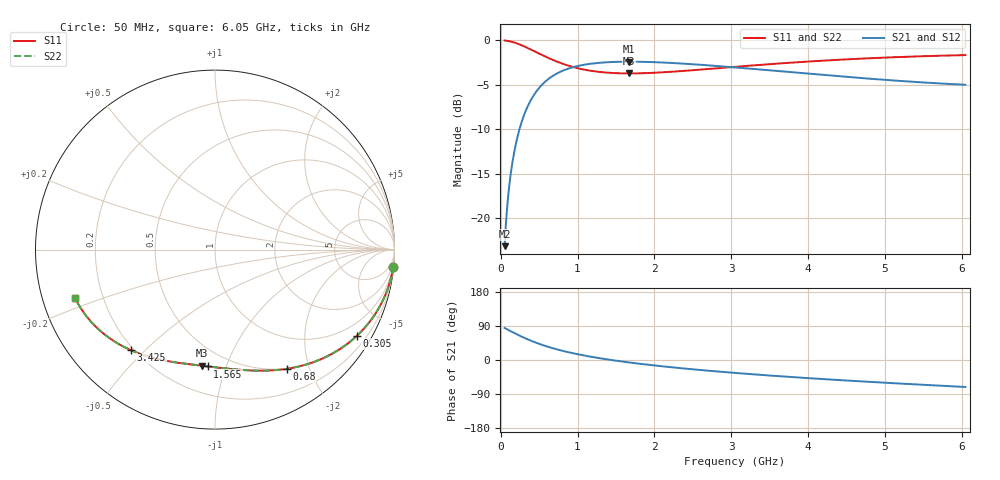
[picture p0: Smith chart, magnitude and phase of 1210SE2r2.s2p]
! AVX Thin Film Operation		Date: August 2001
! Description: Accu-P® Series, Thin Film, SMD, RF Capacitor
! Part Number: 12101J2R2ABT
! 50 MHz  -  6.05 GHz
! Serial Measurements
# mhz S db R 50
!	S11		S21		S12		S22
!	dB	Phase	dB	Phase	dB	Phase	dB	Phase
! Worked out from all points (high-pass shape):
!   401 points, 50 MHz to 6.05 GHz, reference 50 ohm
!   highest |S21| = -2.40 dB at 1.67 GHz (marker M1); lowest = -23.1 dB at 50 MHz (marker M2)
!   |S21| within 3 dB of the highest: 494.6 MHz to end of sweep
!   lowest |S11| = -3.7 dB at 1.67 GHz (marker M3), VSWR 4.74, Z = 18.3 - j41.2 ohm
!   |S11| at or under -10 dB: nowhere
!   |S22| runs from -3.7 to 0.0 dB; largest |S21 - S12| = 0
!   S11 on the Smith chart (normalised r, x): 50 MHz: 1, -21; 305 MHz: 0.53, -3.48; 680 MHz: 0.50, -1.65; 1.565 GHz: 0.38, -0.86; 3.425 GHz: 0.19, -0.45; 6.05 GHz: 0.10, -0.16
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50  -0.02 -5.5  -23.12 84.5  -23.12 84.5  -0.02 -5.5
65  -0.04 -7.1  -20.86 82.9  -20.86 82.9  -0.04 -7.1
110  -0.10 -12.0  -16.38 78.0  -16.38 78.0  -0.10 -12.0
155  -0.20 -16.7  -13.53 73.3  -13.53 73.3  -0.20 -16.7
215  -0.37 -22.8  -10.93 67.2  -10.93 67.2  -0.37 -22.8
305  -0.69 -31.4  -8.36 58.6  -8.36 58.6  -0.69 -31.4
380  -0.99 -38.0  -6.91 52.0  -6.91 52.0  -0.99 -38.0
470  -1.37 -45.1  -5.67 44.9  -5.67 44.9  -1.37 -45.1
560  -1.75 -51.5  -4.79 38.5  -4.79 38.5  -1.75 -51.5
680  -2.22 -59.0  -3.98 30.9  -3.98 30.9  -2.22 -59.0
860  -2.79 -68.5  -3.24 21.5  -3.24 21.5  -2.79 -68.5
1055  -3.24 -76.9  -2.79 13.0  -2.79 13.0  -3.24 -76.9
1280  -3.55 -85.0  -2.53 5.0  -2.53 5.0  -3.55 -85.0
1565  -3.71 -93.6  -2.41 -3.6  -2.41 -3.6  -3.71 -93.6
1670  -3.72 -96.4  -2.40 -6.4  -2.40 -6.4  -3.72 -96.4
2060  -3.62 -105.7  -2.48 -15.7  -2.48 -15.7  -3.62 -105.7
2540  -3.34 -115.3  -2.71 -25.3  -2.71 -25.3  -3.34 -115.3
3050  -2.98 -124.1  -3.05 -34.1  -3.05 -34.1  -2.98 -124.1
3425  -2.73 -129.8  -3.32 -39.9  -3.32 -39.9  -2.73 -129.8
4055  -2.36 -138.5  -3.79 -48.6  -3.79 -48.6  -2.36 -138.5
5060  -1.92 -150.6  -4.48 -60.6  -4.48 -60.6  -1.92 -150.6
6050  -1.67 -161.1  -4.99 -71.2  -4.99 -71.2  -1.67 -161.1
